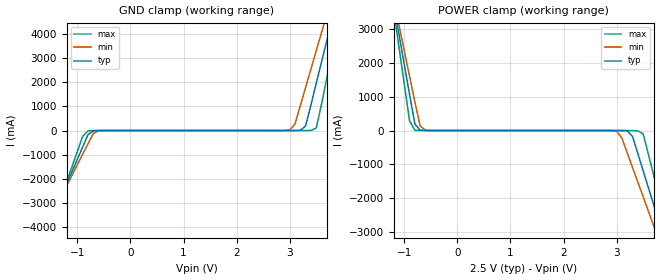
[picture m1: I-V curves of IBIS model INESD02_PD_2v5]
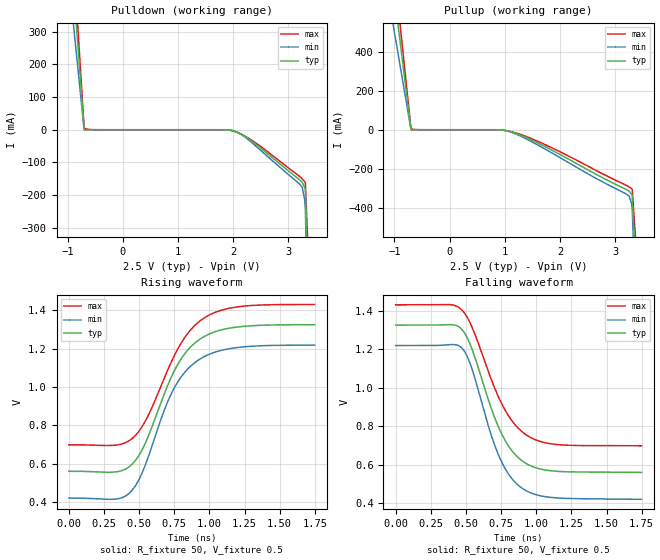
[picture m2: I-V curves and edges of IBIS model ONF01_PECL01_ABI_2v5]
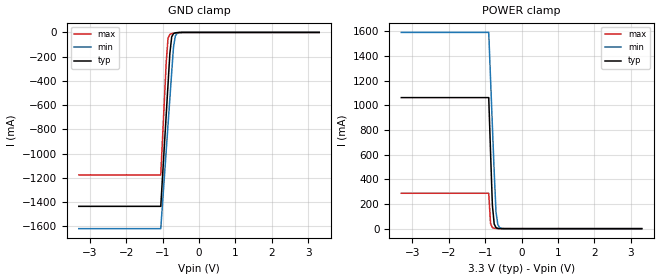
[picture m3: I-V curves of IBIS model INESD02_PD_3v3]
|   This file is an IBIS representation of the   |
|   Integrated Device Technology, Inc.   |
|   ICS843751   |
|   FEMTOCLOCK SAS/SATA CLOCK GENERATOR   |
[IBIS Ver]   4.1
[File name]   843751.ibs
[File Rev]   1.0
[Date]   10 Dec 2009 | Last modified
|   Mar  11 2008 | Generated
[Source]   Originated at Integrated Device Technology, Inc.
[Disclaimer]
IDT hereby grants the user of this IBIS model a non-exclusive,
nontransferable license to use this IBIS model under the following terms.
Before using this IBIS model, the user should read this license.
If the user does not accept these terms,  the IBIS model should be
returned to IDT within 30 days.
   The user is granted this license only to use the IBIS model and
is not granted rights to sell, load, rent, lease or license the IBIS
model in whole or in part, or in modified form to anyone other than
user. User may modify the IBIS model to suit its specific
applications but rights to derivative works and such modifications
shall belong to IDT.
   This IBIS model is provided on an "AS IS" basis and IDT makes
absolutely no warranty with respect to the information contained
herein. IDT DISCLAIMS AND CUSTOMER WAIVES ALL WARRANTIES, EXPRESS
OR IMPLIED, INCLUDING WARRANTIES OF MERCHANTABILITY OR FITNESS FOR
A PARTICULAR PURPOSE. The entire risk as to quality and performance
is with the Customer. ACCORDINGLY, IN NO EVENT SHALL THE COMPANY BE
LIABLE FOR ANY DAMAGES, WHETHER IN CONTRACT OR TORT,INCLUDING ANY
LOST PROFITS OR OTHER INCIDENTAL, CONSEQUENTIAL, EXEMPLARY, OR
PUNITIVE DAMAGES ARISING OUT OF THE USE OR APPLICATION OF THE IBIS
model provided in this package. Further, IDT reserves the right to
make changes without notice to any product herein to improve
reliability, function, or design. IDT does not convey any license
under patent rights or any other intellectual property rights,
including those of third parties.
   IDT is not obligated to provide maintenance or support
for the licensed IBIS model.
[Copyright]   Copyright 2008 by Integrated Device Technology, Inc.
[Component]   ICS843751M
[Manufacturer] Integrated Device Technology, Inc.
[Package]
|SOIC 8 Lead
|   typ   min   max
R_pkg   57.05m   55.5m   58.6m
L_pkg   1.769nH   1.570nH   1.968nH
C_pkg   0.269pF   0.252pF   0.286pF
[Pin] signal_name  model_name   R_pin   L_pin   C_pin
1   XTAL_OUT   NC   58.6m   1.968n   0.286p
2   XTAL_IN   NC   55.5m   1.570n   0.252p
3   SSC_SEL0   INESD02_PD   55.5m   1.570n   0.252p
4   SSC_SEL1   INESD02_PD   56.6m   1.968n   0.286p
5   VCC   POWER   58.6m   1.968n   0.286p
6   Q   ONF01_PECL01_ABI   55.5m   1.570n   0.252p
7   nQ   ONF01_PECL01_ABI   55.5m   1.570n   0.252p
8   VEE   GND   56.6m   1.968n   0.286p
[Diff Pin]  inv_pin  vdiff tdelay_typ tdelay_min  tdelay_max
6   7   NA   0  0  0
[Model Selector] INESD02_PD
INESD02_PD_2v5  Buffer selection for 2v5
INESD02_PD_3v3  Buffer selection for 3v3
[Model Selector] ONF01_PECL01_ABI
ONF01_PECL01_ABI_2v5  Buffer selection for 2v5
ONF01_PECL01_ABI_3v3  Buffer selection for 3v3
| Models and submodels in the file (4): INESD02_PD_2v5 (Input), ONF01_PECL01_ABI_2v5 (Output_ECL), INESD02_PD_3v3 (Input), ONF01_PECL01_ABI_3v3 (Output_ECL)
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[Model] INESD02_PD_2v5
Model_type   Input
Polarity   Non-Inverting
Vinl = 1.4V
Vinh = 1.85V
|   typ   min   max
C_comp   2pF   1.5pF   2.5pF
|   typ   min   max
[Voltage range]  2.5V   2.375V   2.625V
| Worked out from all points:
|   GND clamp passes 1 mA (typ) near -0.55 V on its own axis
|   POWER clamp passes 1 mA (typ) near -0.60 V on its own axis
[GND_clamp]
|Voltage I(typ)   I(min)   I(max)
-2.5V     -8.775A    -7.892A    -10.18A
-1.6V     -4.218A    -4.001A    -4.586A
-900mV    -678.5mA   -979.3mA   -237.6mA
-800mV    -173.9mA   -548.7mA   -10.83mA
-600mV    -1.629mA   -8.74mA    -911.1uA
3V        133.3uA    17.16mA    56.6uA
3.1V      660.9uA    273.5mA    60.87uA
3.3V      191.6mA    1.785A     327.9uA
3.5V      1.949A     3.298A     103.6mA
3.7V      3.723A     4.812A     2.189A
3.9V      5.498A     6.327A     4.369A
5V        15.27A     14.67A     16.38A
[POWER_clamp]
|Voltage   I(typ)   I(min)   I(max)
-2.5V     15.27A     13.72A     17.74A
-1.2V     3.723A     3.866A     3.551A
-1.1V     2.836A     3.109A     2.461A
-900mV    1.063A     1.596A     283.3mA
-800mV    191.6mA    840.1mA    6.189mA
-600mV    660.9uA    8.845mA    114.2uA
3V        -338.1uA   -16.36mA   -12.68uA
3.4V      -678.5mA   -1.518A    -7.183mA
3.5V      -1.183A    -1.95A     -99.52mA
3.7V      -2.195A    -2.813A    -1.324A
4V        -3.712A    -4.109A    -3.188A
5V        -8.775A    -8.432A    -9.404A
[Model] ONF01_PECL01_ABI_2v5
Model_type   Output_ECL
Polarity   Non-Inverting
|   typ   min   max
C_comp   2pF   1.5pF   2.5pF
Vmeas = 0.927V
Rref = 50
Cref = 0
Vref = 0.5V
|   typ   min   max
[Voltage range]   2.5V   2.375V   2.625V
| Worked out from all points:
|   rising waveform, R_fixture 50, V_fixture 0.5: 20-80 % time 275ps typ, 268ps min, 290ps max; typ from 0.56 V to 1.32 V
|   falling waveform, R_fixture 50, V_fixture 0.5: 20-80 % time 232ps typ, 219ps min, 251ps max; typ from 1.32 V to 0.561 V
[Pulldown]
|Voltage   I (typ)   I (min)   I (max)
-2.5V     6.581A     7.946A     5.777A
-1.06V    825.2mA    599mA      978.2mA
-700mV    628.3uA    69.5uA     5.973mA
-552.4mV  32.47uA    1.369uA    245.5uA
2.016V    -3.986mA   -3.148mA   -4.728mA
2.199V    -18.91mA   -20.49mA   -18.13mA
2.429V    -46.47mA   -52.39mA   -42.45mA
3.254V    -161.4mA   -176.1mA   -149.8mA
3.3V      -177mA     -216.4mA   -159.4mA
3.31V     -183.8mA   -242.2mA   -162.5mA
3.648V    -2.082A    -2.875A    -1.578A
5V        -10.5A     -13.61A    -8.61A
[Pullup]
|Voltage   I (typ)   I (min)   I (max)
-2.5V     6.581A     7.946A     5.777A
-1.06V    825.2mA    599mA      978.2mA
-700mV    628.3uA    69.5uA     5.973mA
-552.4mV  32.47uA    1.369uA    245.5uA
915.2mV   -843.2uA   -528uA     -1.018mA
1.144V    -13.7mA    -15.63mA   -12.11mA
1.787V    -94.77mA   -108.1mA   -83.6mA
3.254V    -315.2mA   -340mA     -292.6mA
3.3V      -330.9mA   -380.3mA   -302.4mA
3.31V     -337.7mA   -406.1mA   -305.5mA
3.648V    -2.236A    -3.039A    -1.721A
5V        -10.66A    -13.77A    -8.757A
[Ramp]
|   typ   min   max
dV/dt_r   0.615/0.44n   0.643/0.435n   0.588/0.458n
dV/dt_f   0.613/0.357n   0.642/0.34n   0.586/0.384n
R_load =   50.0000
[Rising Waveform]
R_fixture = 50
V_fixture = 0.5   | VCC_typ - 2V
V_fixture_max = 0.625   | VCC_max - 2V
V_fixture_min = 0.375   | VCC_min - 2V
C_fixture = 0.0p
| Time   typ   min   max
0s        560.2mV    420.6mV    698.3mV
334.6ps   557.1mV    415.2mV    696.8mV
441.4ps   591.2mV    454.2mV    726.2mV
553.6ps   722.4mV    611.7mV    834.8mV
672.7ps   952mV      866.5mV    1.035V
742.7ps   1.073V     985.2mV    1.152V
830.3ps   1.179V     1.081V     1.264V
933.7ps   1.25V      1.146V     1.345V
1.195ns   1.313V     1.206V     1.417V
1.748ns   1.325V     1.219V     1.43V
[Falling Waveform]
R_fixture = 50
V_fixture = 0.5   | VCC_typ - 2V
V_fixture_max = 0.625   | VCC_max - 2V
V_fixture_min = 0.375   | VCC_min - 2V
C_fixture = 0.0p
| Time   typ   min   max
0s        1.325V     1.219V     1.43V
390.6ps   1.328V     1.224V     1.431V
474.7ps   1.299V     1.203V     1.4V
537.8ps   1.211V     1.109V     1.323V
669.2ps   916.1mV    778.4mV    1.064V
737.5ps   786.2mV    641mV      942.3mV
816.3ps   683.5mV    538.3mV    839.4mV
910.9ps   615.1mV    473.2mV    765mV
1.139ns   567.2mV    429.1mV    706.3mV
1.748ns   561mV      421.4mV    699.2mV
[Model] INESD02_PD_3v3
Model_type   Input
Polarity   Non-Inverting
Vinl = 0.80V
Vinh = 2.0V
|   typ   min   max
C_comp   2pF   1.5pF   2.5pF
|   typ   min   max
[Voltage range]  3.3V   3.15V   3.45V
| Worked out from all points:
|   GND clamp passes 1 mA (typ) near -0.56 V on its own axis
|   POWER clamp passes 1 mA (typ) near -0.61 V on its own axis
[GND_clamp]
|Voltage   I(typ)   I(min)   I(max)
-3.3V     -1.436A    -1.62A     -1.176A
-1.05V    -1.436A    -1.62A     -1.176A
-900mV    -678.5mA   -975.1mA   -244mA
-850mV    -426.1mA   -760.1mA   -46.85mA
-800mV    -173.9mA   -545.4mA   -16.11mA
-750mV    -36.96mA   -330.7mA   -9.916mA
-700mV    -9.696mA   -120.2mA   -7.056mA
-650mV    -3.545mA   -29.7mA    -4.857mA
-600mV    -1.629mA   -7.52mA    -3.049mA
-400mV    -52.81uA   -52.52uA   -108.7uA
3.3V      71.13uA    77.43uA    62.11uA
[POWER_clamp]
|Voltage   I(typ)   I(min)   I(max)
-3.3V     1.063A     1.593A     287.3mA
-900mV    1.063A     1.593A     287.3mA
-850mV    620.5mA    1.215A     41.84mA
-800mV    191.6mA    837.5mA    8.757mA
-750mV    37.76mA    460.2mA    3.328mA
-700mV    8.104mA    133.8mA    1.728mA
-650mV    2.076mA    32.66mA    905.3uA
-600mV    678.1uA    8.083mA    443.8uA
-450mV    104.2uA    213.3uA    89.09uA
3.3V      -3.041nA   -3.986uA   0A
